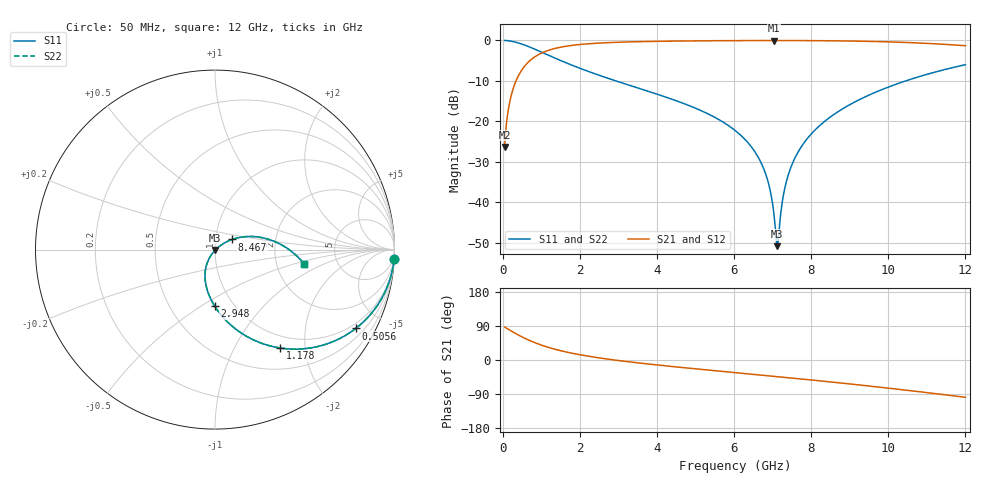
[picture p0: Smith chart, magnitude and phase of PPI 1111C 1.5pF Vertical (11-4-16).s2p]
# GHz S MA R 50
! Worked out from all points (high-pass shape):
!   1601 points, 50 MHz to 12 GHz, reference 50 ohm
!   highest |S21| = -0.03 dB at 7.041 GHz (marker M1); lowest = -26.4 dB at 50 MHz (marker M2)
!   |S21| within 3 dB of the highest: 1.032 GHz to end of sweep
!   lowest |S11| = -50.9 dB at 7.123 GHz (marker M3), VSWR 1.01, Z = 50.2 - j0.199 ohm
!   |S11| at or under -10 dB: 2.93 GHz to 10.46 GHz (7.526 GHz wide, 112 % of centre)
!   |S22| runs from -50.9 to 0.0 dB; largest |S21 - S12| = 0
!   S11 on the Smith chart (normalised r, x): 50 MHz: 1, -37; 505.6 MHz: 0.80, -3.67; 1.178 GHz: 0.80, -1.56; 2.948 GHz: 0.82, -0.57; 8.467 GHz: 1.20, +0.14; 12 GHz: 2.87, -0.59
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0.05  0.9988 -3.1  0.04804 86.9  0.04804 86.9  0.9988 -3.1
0.1470937  0.9901 -9.0  0.1401 81.0  0.1401 81.0  0.9901 -9.0
0.22925  0.9765 -13.9  0.2154 76.1  0.2154 76.1  0.9765 -13.9
0.5055937  0.8989 -29.2  0.4377 60.7  0.4377 60.7  0.8989 -29.2
1.177781  0.6588 -56.4  0.7513 33.6  0.7513 33.6  0.6588 -56.4
2.044156  0.4444 -76.7  0.8944 13.1  0.8944 13.1  0.4444 -76.7
2.947875  0.3143 -90.4  0.9476 -0.7  0.9476 -0.7  0.3143 -90.4
4.038312  0.2136 -103.0  0.9748 -13.5  0.9748 -13.5  0.2136 -103.0
6.025  0.07711 -121.4  0.9942 -33.2  0.9942 -33.2  0.07711 -121.4
6.435781  0.04924 -124.2  0.9958 -37.2  0.9958 -37.2  0.04924 -124.2
6.727062  0.02891 -124.7  0.9965 -40.0  0.9965 -40.0  0.02891 -124.7
6.92125  0.0151 -121.3  0.9967 -41.9  0.9967 -41.9  0.0151 -121.3
7.04075  0.006716 -108.2  0.9968 -43.1  0.9968 -43.1  0.006716 -108.2
7.122906  0.002853 -44.1  0.9968 -43.9  0.9968 -43.9  0.002853 -44.1
7.16025  0.003994 -0.1  0.9967 -44.3  0.9967 -44.3  0.003994 -0.1
7.294688  0.01326 31.7  0.9966 -45.6  0.9966 -45.6  0.01326 31.7
7.436594  0.02403 35.9  0.9963 -47.0  0.9963 -47.0  0.02403 35.9
7.675594  0.04283 36.5  0.9956 -49.4  0.9956 -49.4  0.04283 36.5
8.019156  0.0711 34.5  0.9938 -52.8  0.9938 -52.8  0.0711 34.5
8.467281  0.1102 30.7  0.99 -57.5  0.99 -57.5  0.1102 30.7
10.01331  0.2661 14.7  0.9592 -74.4  0.9592 -74.4  0.2661 14.7
12  0.5009 -8.9  0.8596 -98.3  0.8596 -98.3  0.5009 -8.9
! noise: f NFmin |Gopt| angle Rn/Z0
0.05  0.0007828  0.9556  2.172  0.00397
1.372  0.004083  0.7017  11.7  0.002654
2.701  0.0064  0.6402  19.58  0.003267
4.031  0.008488  0.6107  27.31  0.003831
5.36  0.01052  0.5983  34.72  0.004416
6.682  0.01258  0.5975  41.67  0.005068
8.012  0.01477  0.6058  48.21  0.005841
9.341  0.01716  0.6213  54.32  0.006793
10.67  0.01984  0.6426  60.04  0.007998
12  0.02292  0.6688  65.45  0.009564
